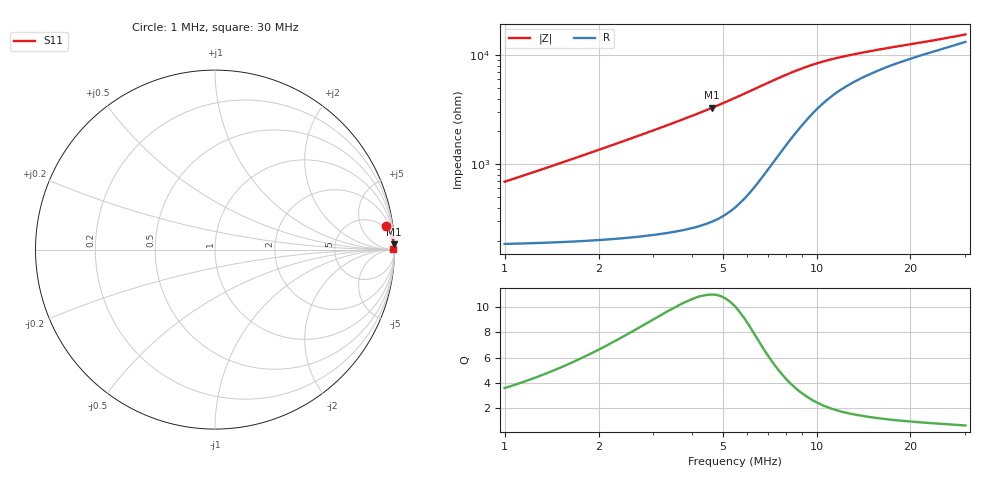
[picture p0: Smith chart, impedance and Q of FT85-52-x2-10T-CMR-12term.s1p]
! ListType=Log
!!FT85-52 x2 10T CMR 12-term
# MHz S RI R 50
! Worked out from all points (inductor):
!   101 points, 1 MHz to 30 MHz, reference 50 ohm
!   read as one part to ground: L = 106 uH near 1 MHz
!   highest Q = 11 at 4.621 MHz (marker M1), where L = 113 uH
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1  0.9528 0.1332
1.107423  0.9605 0.1227
1.226386  0.967 0.1126
1.312713  0.9708 0.1062
1.405116  0.9742 0.1
1.556058  0.9785 0.0912
1.723215  0.9822 0.083
1.908328  0.9852 0.0754
2.113327  0.9877 0.0684
2.262086  0.9892 0.064
2.505087  0.991 0.0579
2.774191  0.9925 0.0523
2.969469  0.9934 0.0488
3.288459  0.9945 0.0439
3.89806  0.9959 0.0366
4.620666  0.9968 0.0301
4.780527  0.9969 0.0289
5.666721  0.9973 0.0234
6.492571  0.9972 0.0195
7.438777  0.9968 0.0162
8.52288  0.9962 0.0135
10.10282  0.9954 0.0108
11.97563  0.9947 0.00894
15.72057  0.9943 0.00679
19.27949  0.9942 0.00554
22.85344  0.9942 0.00465
27.08991  0.9944 0.00382
30  0.9945 0.00333
